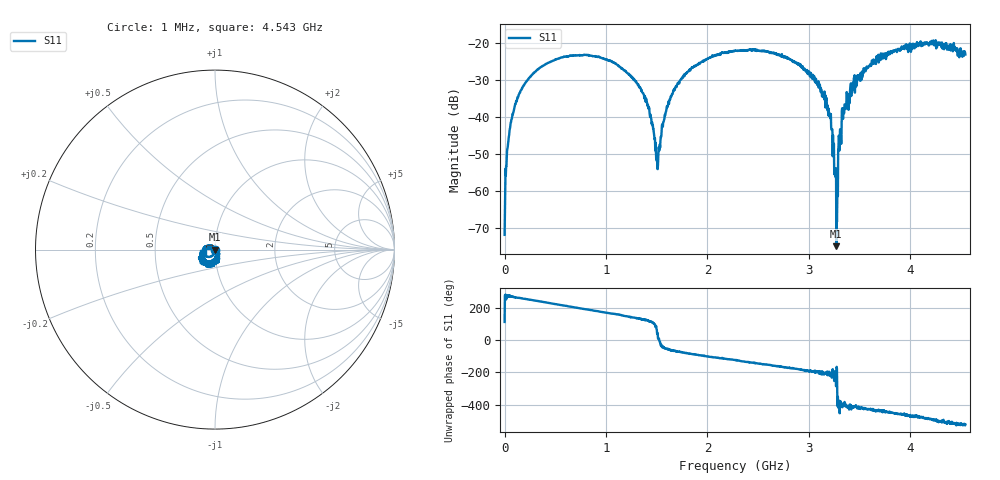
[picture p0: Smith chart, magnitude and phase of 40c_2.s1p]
# HZ S RI R 50
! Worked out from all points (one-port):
!   1515 points, 1 MHz to 4.543 GHz, reference 50 ohm
!   lowest |S11| = -74.9 dB at 3.271 GHz (marker M1), VSWR 1.00, Z = 50 + j0.0116 ohm
!   |S11| at or under -10 dB: start of sweep to end of sweep
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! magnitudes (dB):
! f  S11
! 1 MHz  -71.8
! 28 MHz  -48.5
! 43 MHz  -45.2
! 127 MHz  -34.6
! 298 MHz  -27.8
! 571 MHz  -23.8
! 1.138 GHz  -26.4
! 1.384 GHz  -34.3
! 1.447 GHz  -40.5
! 1.507 GHz  -54.0
! 1.597 GHz  -37.7
! 1.705 GHz  -31.1
! 1.936 GHz  -25.2
! 2.272 GHz  -22.0
! 2.842 GHz  -25.1
! 3.034 GHz  -29.5
! 3.166 GHz  -34.2
! 3.226 GHz  -43.4
! 3.256 GHz  -53.9
! 3.271 GHz  -74.9
! 3.292 GHz  -48.1
! 3.31 GHz  -43.2
! 3.328 GHz  -37.6
! 3.409 GHz  -32.3
! 3.664 GHz  -23.6
! 3.976 GHz  -21.8
! 4.231 GHz  -20.5
! 4.543 GHz  -23.0
